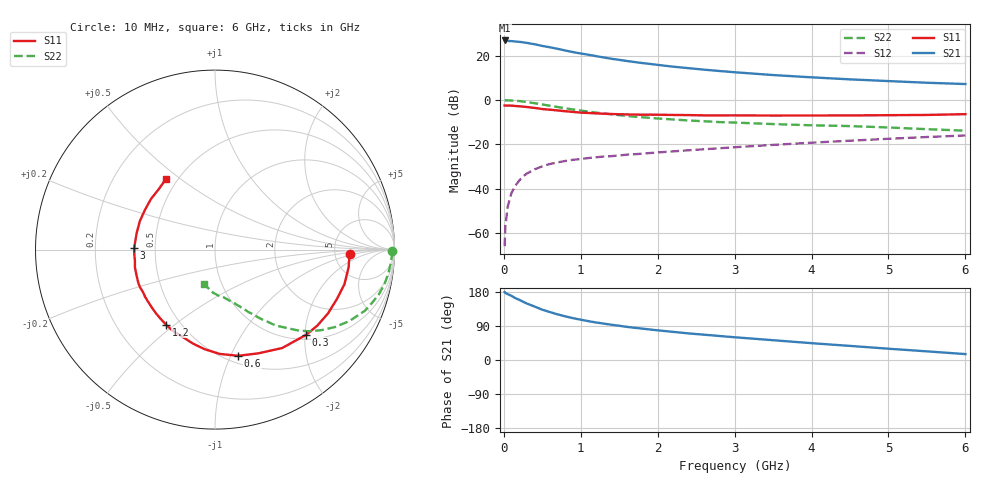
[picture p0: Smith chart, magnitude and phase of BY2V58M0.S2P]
! SIEMENS Small Signal Semiconductors
! BFY420
! Si NPN RF SIEGET Grounded Emitter Transistor in MICRO-X
! VCE = 2.5 V  IC = 8 mA
! Common Emitter S-Parameters:  October  1996
# GHz  S  MA  R  50
!  f  S11  S21  S12  S22
! GHz  MAG  ANG  MAG  ANG  MAG  ANG  MAG  ANG
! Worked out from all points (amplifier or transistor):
!   36 points, 10 MHz to 6 GHz, reference 50 ohm
!   highest |S21| = 26.9 dB at 10 MHz (marker M1)
!   |S21| within 3 dB of that: start of sweep to 584.8 MHz
!   unconditionally stable (mu >= 1): 2.695 GHz to end of sweep
!   at 250 MHz: K = 0.16, MSG = 30.3 dB, |S12| = -34.5 dB
!   at 1.4 GHz: K = 0.68, MSG = 22.0 dB, |S12| = -25.4 dB
!   at 6 GHz: K = 1.11, MAG = 9.6 dB, |S12| = -16.0 dB
!   S11 on the Smith chart (normalised r, x): 10 MHz: 6.94, -0.71; 300 MHz: 1.11, -2.03; 600 MHz: 0.57, -1.07; 1.2 GHz: 0.42, -0.47; 3 GHz: 0.38, +0.01; 6 GHz: 0.43, +0.44
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0.01  0.7505 -1.7  22.17 179.3  0.0005 102.3  0.9857 -0.6
0.02  0.7493 -3.3  22.07 177.0  0.0014 82.2  0.9871 -1.4
0.05  0.751 -7.5  21.56 173.8  0.0039 88.5  0.9836 -3.8
0.1  0.7467 -14.9  21.41 169.3  0.008 82.1  0.9751 -7.8
0.15  0.7333 -21.8  21 163.1  0.0116 77.1  0.9635 -11.6
0.2  0.7232 -29.4  20.62 158.9  0.0152 76.1  0.9466 -15.2
0.3  0.6955 -43.0  19.53 149.0  0.0219 70.0  0.9026 -22.1
0.4  0.6639 -55.7  18.19 141.0  0.0272 64.8  0.8481 -28.0
0.5  0.6263 -67.4  16.68 132.7  0.0318 60.2  0.795 -32.9
0.6  0.6053 -77.8  15.52 126.4  0.036 56.7  0.7425 -37.2
0.7  0.5815 -87.5  14.33 120.4  0.0391 54.5  0.6947 -40.9
0.8  0.5582 -95.8  13.12 115.1  0.0421 51.3  0.6501 -44.0
0.9  0.5383 -103.1  12.11 110.3  0.0447 49.9  0.6112 -46.3
1.1  0.5104 -117.5  10.53 102.5  0.049 47.8  0.5483 -50.8
1.2  0.4988 -123.2  9.801 99.0  0.0509 47.0  0.5201 -52.6
1.6  0.4725 -142.3  7.61 87.4  0.0584 45.0  0.4361 -58.3
2.2  0.4601 -162.0  5.671 74.2  0.0692 44.2  0.3642 -64.7
3  0.4507 179.0  4.243 60.0  0.0858 42.2  0.3097 -71.6
3.5  0.4461 168.1  3.666 52.2  0.0969 40.5  0.2863 -75.9
4.5  0.4485 150.5  2.929 37.2  0.1206 35.1  0.2579 -85.4
5.5  0.4606 132.4  2.457 22.8  0.1461 28.0  0.2196 -99.2
6  0.4797 124.7  2.297 15.6  0.1584 23.9  0.2031 -108.2
